(* Logix 5000 Routine export MainRoutine; software revision 20.04 *)

TYPE Segment_Status :
STRUCT
   Speed_pulse_status : BOOL; {access Read Only}
   Exists : BOOL; {access Read Only}
   Group_number : INT; {access Read Only}
END_STRUCT
END_TYPE

VAR_GLOBAL   (* controller tags *)
   Trigger_Group_Write : DINT;
   Status_of_Segments : Segment_Status[50]; {access Read Only}
   msg_Group : MESSAGE;
        MessageParameters(MessageType := CIP Generic, RequestedLength := 2, ConnectedFlag := 2, ConnectionPath := segFORCE, ServiceCode := 16#0010, ObjectType := 16#0087, TargetObject := 1, AttributeNumber := 16#0001, LocalElement := Group_Mode)
   Group_Mode : DINT;
END_VAR

PROGRAM MainProgram

ROUTINE MainRoutine   (* ladder *)
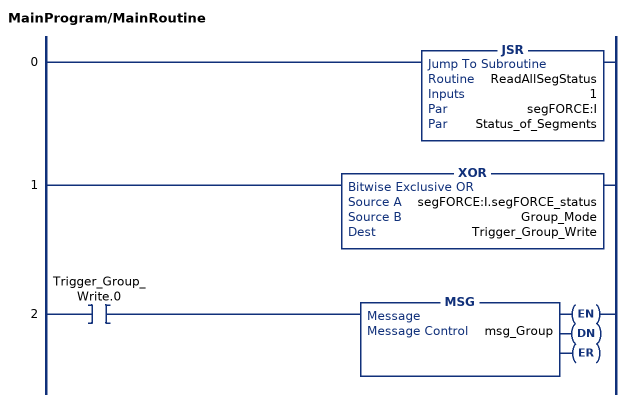
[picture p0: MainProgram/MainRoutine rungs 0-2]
   0: JSR(ReadAllSegStatus,1,segFORCE:I,Status_of_Segments);
   1: XOR(segFORCE:I.segFORCE_status,Group_Mode,Trigger_Group_Write);
   2: XIC(Trigger_Group_Write.0)MSG(msg_Group);
END_ROUTINE
END_PROGRAM
